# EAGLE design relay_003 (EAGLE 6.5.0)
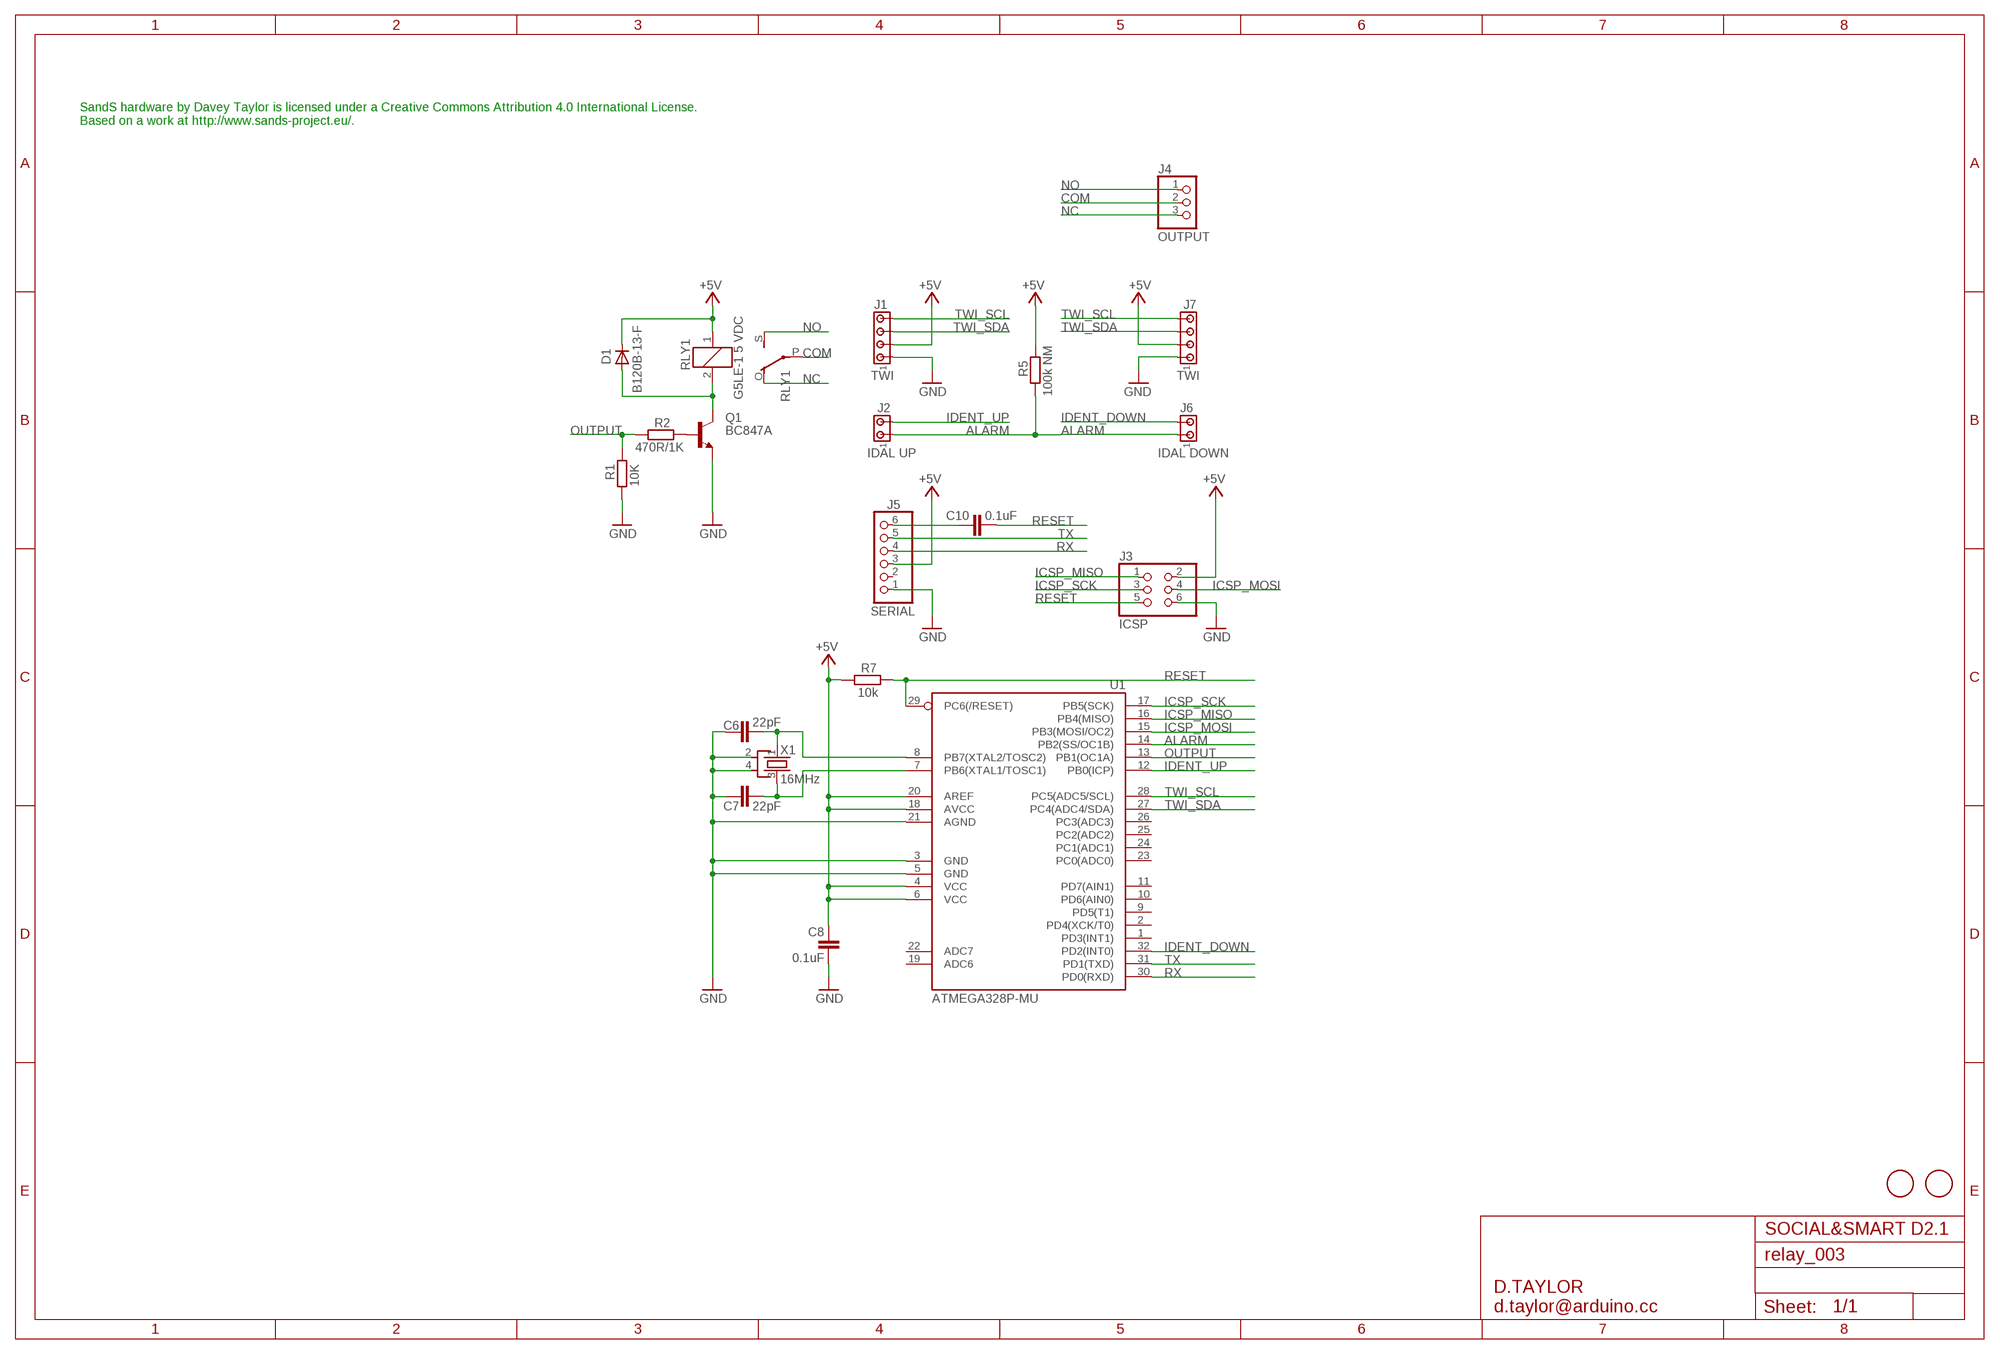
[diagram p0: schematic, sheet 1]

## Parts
C6  22pF  C-EUC0603  [C0603]
C7  22pF  C-EUC0603  [C0603]
C8  0.1uF  C-EUC0603  [C0603]
C10  0.1uF  C-EUC0603  [C0603]
D1  B120B-13-F  DIODE-SMB  [SMB]
J1  TWI  MTA04-100  [10X04MTA]
J2  IDAL UP  MTA02-100  [10X02MTA]
J3  ICSP  PINHD-2X3  [2X03]
J4  OUTPUT  MKDS_1,5/3-5,08  [MKDS1,5/3-5,08]
J5  SERIAL  PINHD-1X6  [1X06]
J6  IDAL DOWN  MTA02-100  [10X02MTA]
J7  TWI  MTA04-100  [10X04MTA]
Q1  BC847A  BC847ASMD  [SOT23]
R1  10K  R-EU_R0603  [R0603]
R2  470R/1K  R-EU_R0603  [R0603]
R5  100k NM  R-EU_R0603  [R0603]
R7  10k  R-EU_R0603  [R0603]
RLY1  G5LE-1 5 VDC  G5LE  [G5LE]
U1  ATMEGA328P-MU  [MLF32-M1-A]
U$5  FIDUCIALMOUNT  [FIDUCIA-MOUNT]
U$6  FIDUCIALMOUNT  [FIDUCIA-MOUNT]
X1  16MHz  CRYSTAL-KX7  [XTAL-3.2-2.5]

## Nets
+5V: C8.1 D1.C J1.2 J3.2 J5.3 J7.2 R5.2 R7.1 RLY1.1 U1.4(VCC) U1.6(VCC) U1.18(AVCC) U1.20(AREF)
ALARM: J2.1 J6.1 R5.1 U1.14(PB2(SS/OC1B))
COM [PWR]: J4.2 RLY1.P(2:P)
GND: C6.1 C7.1 C8.2 J1.1 J3.6 J5.1 J7.1 Q1.2(E) R1.2 U1.3(GND) U1.5(GND) U1.21(AGND) X1.2(SH1) X1.4(SH2)
ICSP_MISO: J3.1 U1.16(PB4(MISO))
ICSP_MOSI: J3.4 U1.15(PB3(MOSI/OC2))
ICSP_SCK: J3.3 U1.17(PB5(SCK))
IDENT_DOWN: J6.2 U1.32(PD2(INT0))
IDENT_UP: J2.2 U1.12(PB0(ICP))
N$2: D1.A Q1.3(C) RLY1.2
N$4: Q1.1(B) R2.1
N$6: C6.2 U1.8(PB7(XTAL2/TOSC2)) X1.1(X1)
N$7: C7.2 U1.7(PB6(XTAL1/TOSC1)) X1.3(X2)
N$9: C10.1 J5.6
NC [PWR]: J4.3 RLY1.O(2:O)
NO [PWR]: J4.1 RLY1.S(2:S)
OUTPUT: R1.1 R2.2 U1.13(PB1(OC1A))
RESET: C10.2 J3.5 R7.2 U1.29(PC6(/RESET))
RX: J5.4 U1.30(PD0(RXD))
TWI_SCL: J1.4 J7.4 U1.28(PC5(ADC5/SCL))
TWI_SDA: J1.3 J7.3 U1.27(PC4(ADC4/SDA))
TX: J5.5 U1.31(PD1(TXD))
Unconnected: J5.2 U1.1(PD3(INT1)) U1.2(PD4(XCK/T0)) U1.9(PD5(T1)) U1.10(PD6(AIN0)) U1.11(PD7(AIN1)) U1.19(ADC6) U1.22(ADC7) U1.23(PC0(ADC0)) U1.24(PC1(ADC1)) U1.25(PC2(ADC2)) U1.26(PC3(ADC3))

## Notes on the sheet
- SandS hardware by Davey Taylor is licensed under a Creative Commons Attribution 4.0 International License.
  Based on a work at http://www.sands-project.eu/.
- SOCIAL&SMART D2.1
- D.TAYLOR
  d.taylor@arduino.cc

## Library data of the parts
C6-C8 C10 = rcl:C-EU: CAPACITOR, European symbol
D1 = diode:DIODE-: DIODE
J1 J7 = con-amp:MTA04-100: AMP connector
J2 J6 = con-amp:MTA02-100: AMP connector
J3 = pinhead:PINHD-2X3: PIN HEADER
J4 = d_taylor:MKDS_1,5/3-5,08: MKDSN 1,5/ 3-5,08 Printklemme Nennstrom: 13,5 A Nennspannung: 250 V Rastermaß: 5,08 mm Polzahl: 3 Anschlussart: Schraubanschluss Montage: Löten Anschlussrichtung Leiter/Platine: 0 ° Artikelnummer: 1729131 Source: http://eshop.phoenixcontact.com .. 1729131.pdf; MPN: SMKDSN1,5/3-5,08; OC_FARNELL: 1792904; OC_NEWARK: 70R0299
J5 = pinhead:PINHD-1X6: PIN HEADER
Q1 = transistor-npn:BC847*: NPN Transistor
R1 R2 = SmartPrj:R-EU_: RESISTOR, European symbol
R5 R7 = rcl:R-EU_: RESISTOR, European symbol
RLY1 = relay:G5LE: RELAY 1 x switch, 10 A/120 V AC, 8 A/30 V DC, Omron; OC_FARNELL: unknown; OC_NEWARK: unknown
U1 = d_taylor:ATMEGA*: MICROCONTROLLER 8 Kbytes FLASH 1 kbytes SRAM 512 bytes EEPROM USART 6-channel 10 bit ADC 2-channel 8 bit ADC Source: avr.lbr
U$5 U$6 = SmartPrj:FIDUCIALMOUNT
X1 = d_taylor:CRYSTAL-KX7

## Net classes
1 PWR: width 0.406 mm, clearance 0.61 mm

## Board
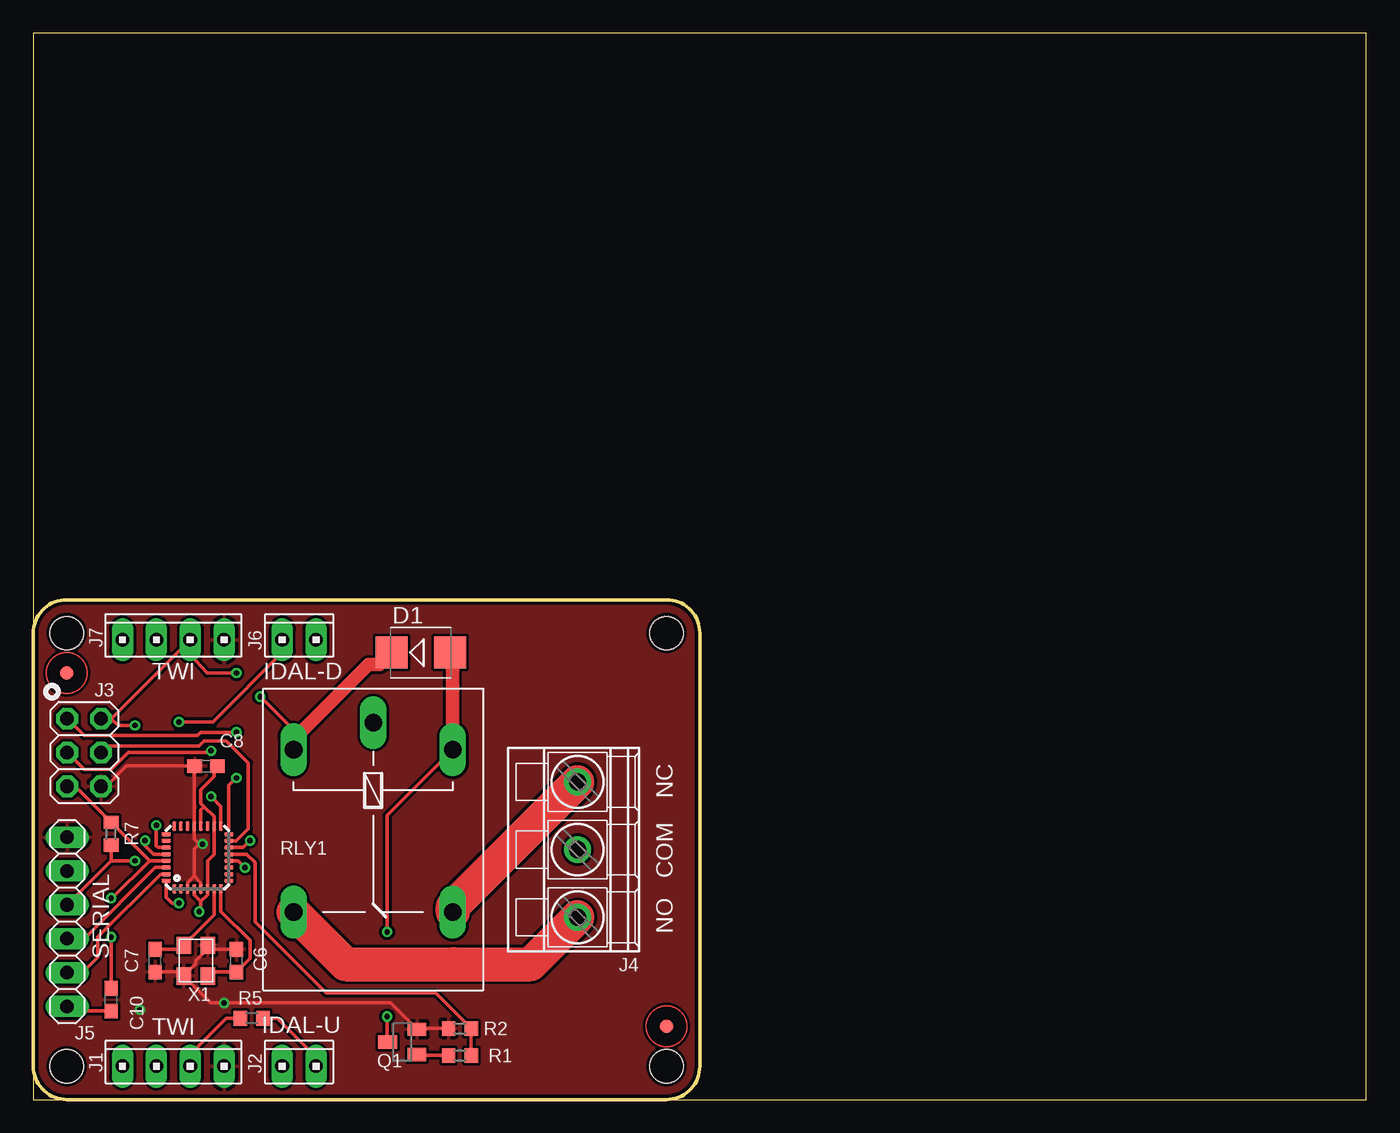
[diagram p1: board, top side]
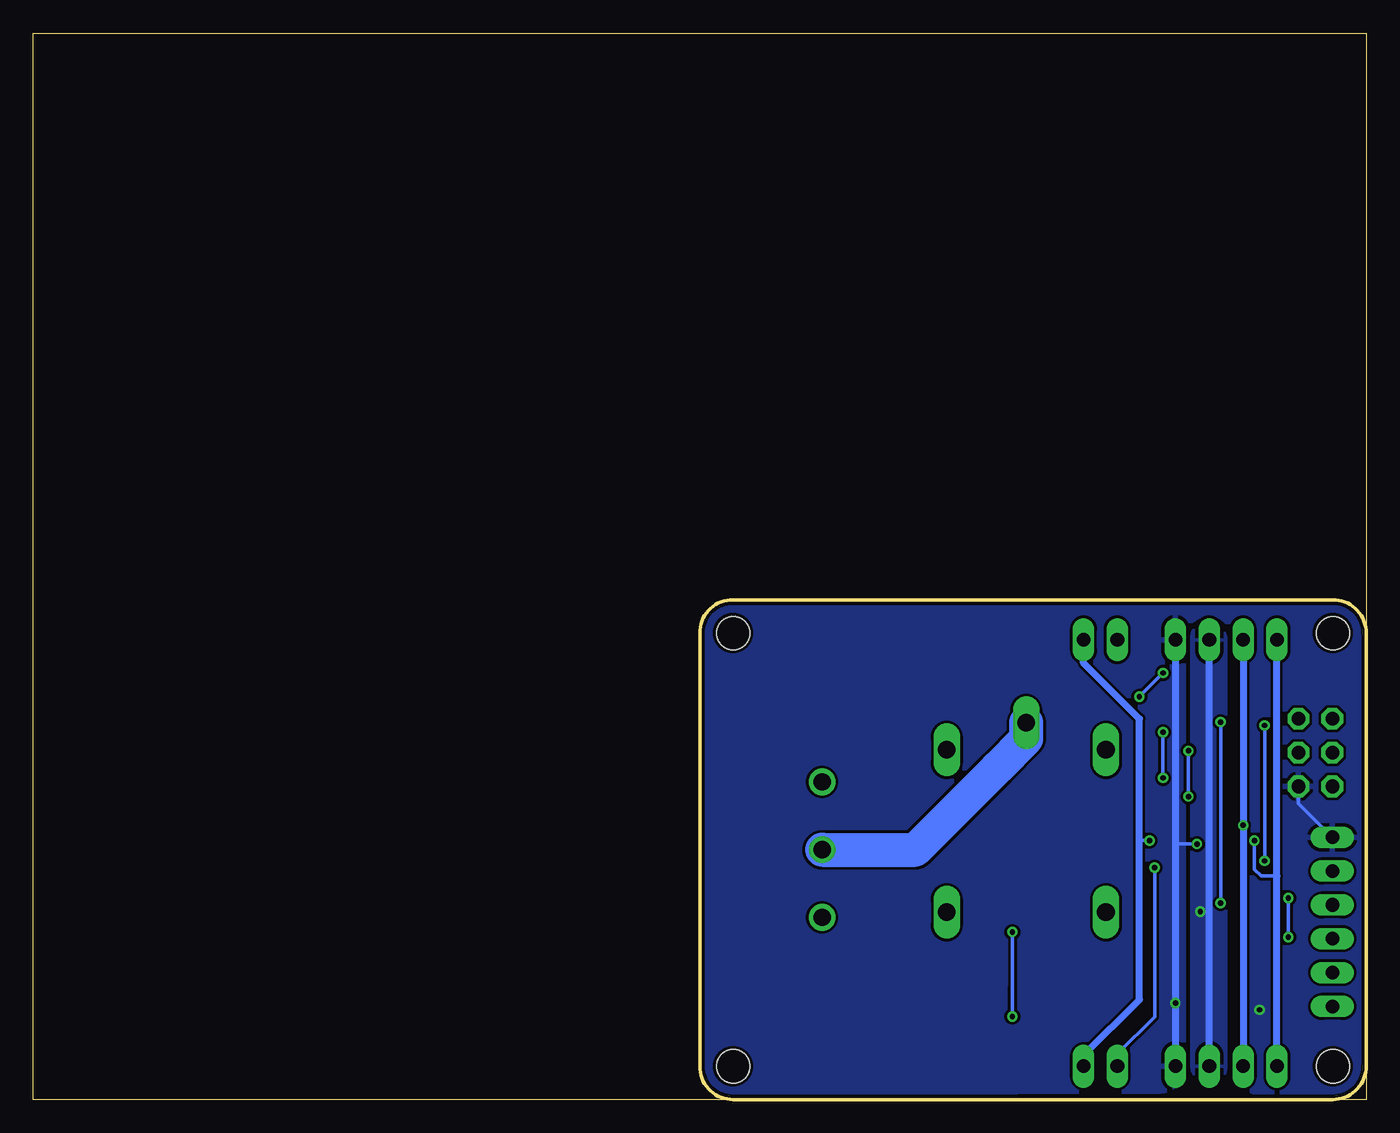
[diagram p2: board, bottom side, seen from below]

Size 100 x 80 mm. Coordinates in mm from the lower left corner, seen from the top.
Outline: 0,35 0,80 100,80 100,0 0,0 0,35
Outline: 0,35 arc-90 2.5,37.5 47.5,37.5 arc-90 50,35 50,2.5 arc-90 47.5,0 2.5,0 arc-90 0,2.5 0,35
Copper layers (1*16): Top 0.035mm / dielectric 1.5mm / Bottom 0.035mm
Design rules "smartprj-mini *": minimum track width 8mil, minimum drill 10mil, track to track 8mil, track to pad 8mil, pad to pad 0.200659375mm, via to via 8mil, smd to smd 4mil, copper to edge 10mil, drill to drill 8mil, minimum pad ring 12mil, minimum via ring 7mil, stop-mask expansion 2mil, vias tented up to drill 20mil, thermal gap 10mil
Holes 2.5 mm at 2.5,35 2.5,2.5 47.5,2.5 47.5,35

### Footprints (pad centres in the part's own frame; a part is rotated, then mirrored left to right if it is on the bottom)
C0603 = smd 1.1 x 1: 1 -0.85,0; 2 0.85,0
SMB = smd 2.4 x 2.4: A 2.2,0; C -2.2,0
10X04MTA = drill 1.016 long: 1 3.81,0; 2 1.27,0; 3 -1.27,0; 4 -3.81,0
10X02MTA = drill 1.016 long: 1 1.27,0; 2 -1.27,0
2X03 = drill 1.016 octagon: 1 -2.54,-1.27; 2 -2.54,1.27; 3 0,-1.27; 4 0,1.27; 5 2.54,-1.27; 6 2.54,1.27
MKDS1,5/3-5,08 = drill 1.3 pad 2: 1 -5.08,0; 2 0,0; 3 5.08,0
1X06 = drill 1.016 long: 1 -6.35,0; 2 -3.81,0; 3 -1.27,0; 4 1.27,0; 5 3.81,0; 6 6.35,0
SOT23 = smd 1 x 1.4: 1 -0.95,-1.1; 2 0.95,-1.1; 3 0,1.1
R0603 = smd 1 x 1.1: 1 -0.85,0; 2 0.85,0
G5LE = drill 1.321 long: 1 -7.493,-5.969; 2 -7.493,5.969; O 4.699,5.969; P -9.525,0; S 4.699,-5.969
MLF32-M1-A = smd 0.7 x 0.3: 1 -2.35,1.75; 2 -2.35,1.25; 3 -2.35,0.75; 4 -2.35,0.25; 5 -2.35,-0.25; 6 -2.35,-0.75; 7 -2.35,-1.25; 8 -2.35,-1.75; 17 2.35,-1.75; 18 2.35,-1.25; 19 2.35,-0.75; 20 2.35,-0.25; 21 2.35,0.25; 22 2.35,0.75; 23 2.35,1.25; 24 2.35,1.75 | smd 0.3 x 0.7: 9 -1.75,-2.35; 10 -1.25,-2.35; 11 -0.75,-2.35; 12 -0.25,-2.35; 13 0.25,-2.35; 14 0.75,-2.35; 15 1.25,-2.35; 16 1.75,-2.35; 25 1.75,2.35; 26 1.25,2.35; 27 0.75,2.35; 28 0.25,2.35; 29 -0.25,2.35; 30 -0.75,2.35; 31 -1.25,2.35; 32 -1.75,2.35
FIDUCIA-MOUNT = smd 1.016 x 1.016: P$1 0,0
XTAL-3.2-2.5 = smd 1.3 x 1.1: 1 -1.15,-0.9; 2 1.15,-0.9; 3 1.15,0.9; 4 -1.15,0.9

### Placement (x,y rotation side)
C6  15.24,10.41 270 top
C7  9.14,10.41 90 top
C8  12.95,25.02 180 top
C10  5.84,7.49 90 top
D1  29.08,33.53 0 top
J1  10.5,2.5 0 top
J2  19.94,2.5 0 top
J3  3.81,26.04 270 top
J4  40.83,18.75 90 top
J5  2.54,13.34 270 top
J6  19.94,34.5 0 top
J7  10.5,34.5 0 top
Q1  27.69,4.32 90 top
R1  32,5.33 180 top
R2  32,3.3 0 top
R5  16.38,6.1 180 top
R7  5.84,19.94 90 top
RLY1  25.5,18.75 270 top
U1  12.32,18.16 90 top
U$5  2.5,32 0 top
U$6  47.5,5.5 0 top
X1  12.19,10.41 90 top

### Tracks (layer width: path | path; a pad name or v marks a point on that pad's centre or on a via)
+5V  (via drill 0.41 pad 0.61)
  Top 0.254: 12.57,14.86 13.07,15.36 U1.6 13.07,17.89 13.57,18.39 U1.18 13.57,21.23 12.83,21.97 | 12.57,14.86 12.07,15.36 U1.4 | C8.1 13.57,24.78 13.57,24.24 12.57,23.24 12.57,22.23 12.83,21.97 | R7.1 5.84,17.91 | 5.84,17.91 J5.3 | J1.2 11.77,3.39 14.48,6.1 R5.2 | 12.57,14.86 12.57,14.22 v12.45,14.1 | 5.84,28.57 J7.2 11.77,33.4 13.04,32 v15.24,32 | 5.84,28.57 J3.2 | 5.84,17.91 v7.62,17.91 | v7.62,28.07 6.35,28.07 5.84,28.57 | RLY1.1 19.53,27.71 v17.02,30.23 | U1.20 12.57,21.71 12.83,21.97
  Top 1.016: RLY1.1 19.53,27.02 25.15,32.64 25.99,32.64 D1.C
  Bottom 0.254: v12.45,14.1 11.77,14.1 | v7.62,17.91 v7.62,28.07 | v17.02,30.23 v15.24,32
  Bottom 0.508: J1.2 11.77,14.1 J7.2
  pour Bottom: 13.08,34.67 arc90 11.94,35.81 11.81,35.81 arc90 10.54,34.54 10.54,2.54 10.54,2.41 arc90 11.68,1.27 11.81,1.27 arc90 13.08,2.54
ALARM  (via drill 0.41 pad 0.61)
  Top 0.254: J2.1 21.21,3.17 18.29,6.1 R5.1 | U1.14 15.74,18.91 v16.26,19.43
  Bottom 0.254: v16.26,19.43 17.02,19.43
  Bottom 0.508: J2.1 21.21,3.3 17.02,7.49 17.02,19.43 17.02,28.57 21.21,32.77 J6.1
COM
  Bottom 2.54: J4.2 33.83,18.75 27.69,24.89 25.5,27.08 RLY1.P
GND  (via drill 0.41, 0.41 pad 0.61)
  Top 0.254: X1.4 10.99,9.56 C7.1 | X1.2 13.39,11.26 C6.1 | X1.2 13.08,11.43 | X1.4 12.19,10.16 12.19,10.41 13.09,11.31 X1.2 | U1.3 11.57,16.27 12.06,16.76 | 12.06,16.76 12.57,16.26 U1.5 | 12.06,16.76 12.07,16.89 12.06,18.8 12.45,19.18 | 12.45,19.18 12.07,19.55 U1.21 12.07,24.98 C8.2 6.99,25.02 5.46,23.5 J3.6 | R1.2 28.85,5.33 Q1.2 26.82,7.24 v14.31,7.24 13.32,7.24 X1.4 | 12.45,19.18 v12.7,19.18
  Bottom 0.254: J3.6 5.08,22.23 J5.1 | v12.7,19.18 14.31,19.18
  Bottom 0.508: J7.1 14.31,19.18 14.31,8.26 v14.31,7.24 J1.1
  other vias: 8,6.73
  pour Top: 0.5,35 arc-90 2.5,37 47.5,37 arc-90 49.5,35 49.5,2.5 arc-90 47.5,0.5 2.5,0.5 arc-90 0.5,2.5
  pour Bottom: 0.5,35 arc-90 2.5,37 47.5,37 arc-90 49.5,35 49.5,2.5 arc-90 47.5,0.5 15.49,0.64 arc-90 13.72,2.41 13.72,34.42 arc90 11.81,36.45 arc90 9.91,34.54 9.91,2.54 arc-90 7.87,0.5 2.5,0.5 arc-90 0.5,2.5
ICSP_MISO  (via drill 0.41)
  Top 0.254: U1.16 14.67,23.56 v15.24,24.13 | v15.24,27.56 12.57,27.56 12.32,27.3 3.81,27.3 J3.1
  Bottom 0.254: v15.24,24.13 v15.24,27.56
ICSP_MOSI
  Top 0.254: U1.15 15.22,19.41 16.13,20.32 16.13,25.27 14.48,26.92 12.83,26.92 12.45,26.54 5.59,26.54 J3.4
ICSP_SCK  (via drill 0.41, 0.41 pad 0.61)
  Top 0.254: U1.17 14.07,22 v13.34,22.73 | v13.34,26.16 13.21,26.04 7.11,26.04 5.84,24.77 3.81,24.77 J3.3
  Bottom 0.254: v13.34,22.73 v13.34,26.16
IDENT_DOWN  (via drill 0.41 pad 0.61)
  Top 0.254: J6.2 18.67,33.53 13.51,28.32 v10.92,28.32 | U1.32 9.97,15.18 10.41,14.73 v10.92,14.73
  Bottom 0.254: v10.92,28.32 v10.92,14.73
IDENT_UP  (via drill 0.41 pad 0.61)
  Top 0.254: v15.88,17.4 15.36,17.91 U1.12
  Bottom 0.254: J2.2 18.67,3.43 15.88,6.22 v15.88,17.4
N$2  (via drill 0.41 pad 0.61)
  Top 0.254: RLY1.2 26.54,21.32 v26.54,12.57 | Q1.3 26.54,4.36 v26.54,6.22
  Top 1.016: RLY1.2 31.47,33.34 D1.A
  Bottom 0.254: v26.54,12.57 26.54,8.51 | 26.54,8.51 v26.54,6.22 26.54,8.51
N$4
  Top 0.254: R2.1 28.85,3.3 Q1.1
N$6
  Top 0.254: X1.1 13.39,9.56 C6.2 16.26,10.58 16.26,11.94 14.07,14.12 U1.8
N$7
  Top 0.254: C7.2 10.99,11.26 X1.3 13.57,13.84 U1.7
N$9
  Top 0.254: J5.6 2.88,6.64 C10.1
NC
  Top 2.54: RLY1.O 31.47,14.47 J4.3
NO
  Top 2.54: RLY1.S 23.42,10.16 31.5,10.16 37.31,10.16 J4.1
OUTPUT
  Top 0.254: U1.13 16.01,18.41 16.64,17.78 16.64,13.34 21.97,8 30.19,8 R1.1 R2.2
RESET  (via drill 0.41 pad 0.61)
  Top 0.254: J3.5 3.14,23.5 R7.2 8.72,17.91 | U1.29 8.72,17.91 | v5.84,12.19 C10.2 | v5.84,15.11 5.92,15.11 8.72,17.91
  Bottom 0.254: v5.84,15.11 v5.84,12.19
RX
  Top 0.254: U1.30 9.16,17.41 3.81,12.06 J5.4
TWI_SCL  (via drill 0.41 pad 0.61)
  Top 0.254: 8.38,19.05 v8.38,19.43 8.38,19.05 | U1.28 9.02,18.41 8.38,19.05
  Bottom 0.254: v8.38,19.43 8.38,17.27 7.87,16.76 6.69,16.76
  Bottom 0.508: J1.4 6.69,16.76 J7.4
TWI_SDA  (via drill 0.41 pad 0.61)
  Top 0.254: U1.27 9.37,18.91 9.23,19.05 v9.23,20.57
  Bottom 0.508: J7.3 v9.23,20.57 J1.3
TX
  Top 0.254: U1.31 9.54,16.91 4.83,12.19 4.83,10.67 3.68,9.53 J5.5

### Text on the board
tPlace: TWI | IDAL-D | NC | COM | NO | SERIAL | TWI | IDAL-U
